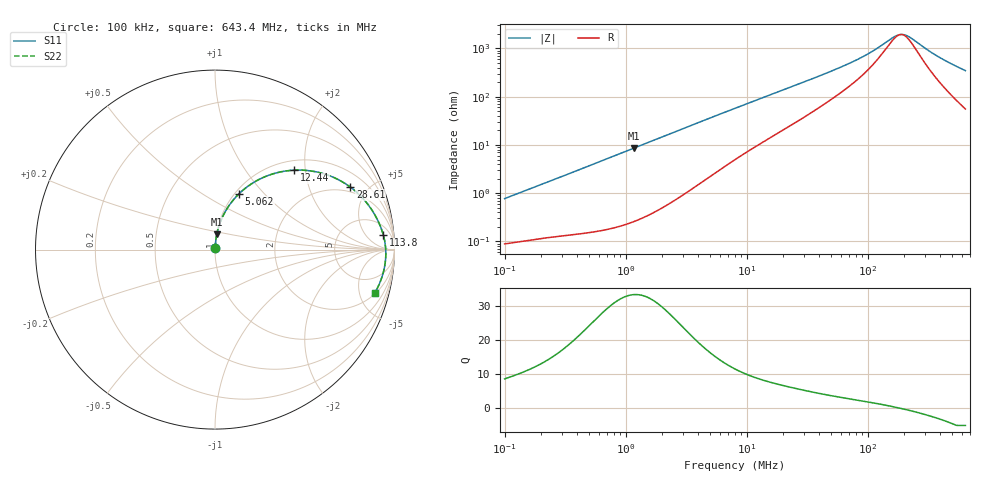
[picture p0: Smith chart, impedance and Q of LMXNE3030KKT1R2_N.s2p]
! LMXNE3030KKT1R2_N  S-PARAMETER MODEL  ( General Type )
! Model Generated by TAIYO YUDEN Corporation (http://www.ty-top.com)
! Version 1.0
! TAIYO YUDEN Control No. 191023NI43SB-FBB
! Copyright(c) 2019 TAIYO YUDEN CO.,LTD. All Rights Reserved.
! Product Description (link to TY-COMPAS)
! https://ds.yuden.co.jp/TYCOMPAS/or/detail?pn=LMXNE3030KKT1R2NN&u=M
! Products Name : Inductors
! Characteristics :
!  Inductance : 1.2 uH , SRF(min) : 120 MHz , DC Resistance(max) : 0.078 Ohm
!  Rated Current : Saturation :1700 mA , Temp Rise : 1480 mA
!  Case Size : 3.0 x 3.0 / 0.118 x 0.118 [mm/inch] , Thickness : 1 / 0.039 [mm/inch]
!  (Conditions: Temperature = 25 degC , DC Bias Current/Voltage = 0A / 0V)
! External Node Assignments :
!  1  o---GGG---o  2
! GND o---------o GND
! Frequency Range : 0.1MHz  -  643.381979MHz  [ 402 STEP ]
# MHz S RI R 50
! Freq[MHz].  S11 Real  S11 Imag  S21 Real  S21 Imag  S12 Real  S12 Imag  S22 Real  S22 Imag
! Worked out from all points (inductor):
!   401 points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, 100 kHz to 643.4 MHz, reference 50 ohm
!   read as one part in series: L = 1.21 uH near 104.5 kHz
!   highest Q = 33.3 at 1.165 MHz (marker M1), where L = 1.17 uH
!   self-resonance near 188.2 MHz
!   S11 on the Smith chart (normalised r, x): 100 kHz: 1.00, +0.02; 5.062 MHz: 1.05, +0.74; 12.44 MHz: 1.20, +1.74; 28.61 MHz: 1.70, +3.82; 113.8 MHz: 11, +16; 643.4 MHz: 2.11, -6.86
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0.1  0.000948 0.00768  0.9991 -0.00768  0.9991 -0.00768  0.000948 0.00768
0.434429  0.00248 0.0321  0.9975 -0.0321  0.9975 -0.0321  0.00248 0.0321
1.165122  0.00982 0.0847  0.9902 -0.0847  0.9902 -0.0847  0.00982 0.0847
1.887283  0.0232 0.1349  0.9768 -0.1349  0.9768 -0.1349  0.0232 0.1349
3.264874  0.0629 0.2215  0.9371 -0.2215  0.9371 -0.2215  0.0629 0.2215
5.061623  0.1341 0.3112  0.8659 -0.3112  0.8659 -0.3112  0.1341 0.3112
8.02111  0.2664 0.4009  0.7336 -0.4009  0.7336 -0.4009  0.2664 0.4009
12.43535  0.4405 0.4426  0.5595 -0.4426  0.5595 -0.4426  0.4405 0.4426
18.05169  0.5959 0.4253  0.4041 -0.4253  0.4041 -0.4253  0.5959 0.4253
28.60635  0.7532 0.349  0.2468 -0.349  0.2468 -0.349  0.7532 0.349
34.846  0.8028 0.3071  0.1972 -0.3071  0.1972 -0.3071  0.8028 0.3071
48.41396  0.8632 0.2368  0.1368 -0.2368  0.1368 -0.2368  0.8632 0.2368
70.2798  0.9065 0.1637  0.0935 -0.1637  0.0935 -0.1637  0.9065 0.1637
91.42912  0.9263 0.1171  0.0737 -0.1171  0.0737 -0.1171  0.9263 0.1171
113.8404  0.938 0.0806  0.062 -0.0806  0.062 -0.0806  0.938 0.0806
151.3811  0.9476 0.0348  0.0524 -0.0348  0.0524 -0.0348  0.9476 0.0348
180.4018  0.9507 0.00684  0.0493 -0.00684  0.0493 -0.00684  0.9507 0.00684
192.6657  0.9514 -0.00375  0.0486 0.00375  0.0486 0.00375  0.9514 -0.00375
210.3241  0.9518 -0.018  0.0482 0.018  0.0482 0.018  0.9518 -0.018
380.155  0.9387 -0.1237  0.0613 0.1237  0.0613 0.1237  0.9387 -0.1237
505.5173  0.9187 -0.1843  0.0813 0.1843  0.0813 0.1843  0.9187 -0.1843
643.382  0.8903 -0.2417  0.1097 0.2417  0.1097 0.2417  0.8903 -0.2417
